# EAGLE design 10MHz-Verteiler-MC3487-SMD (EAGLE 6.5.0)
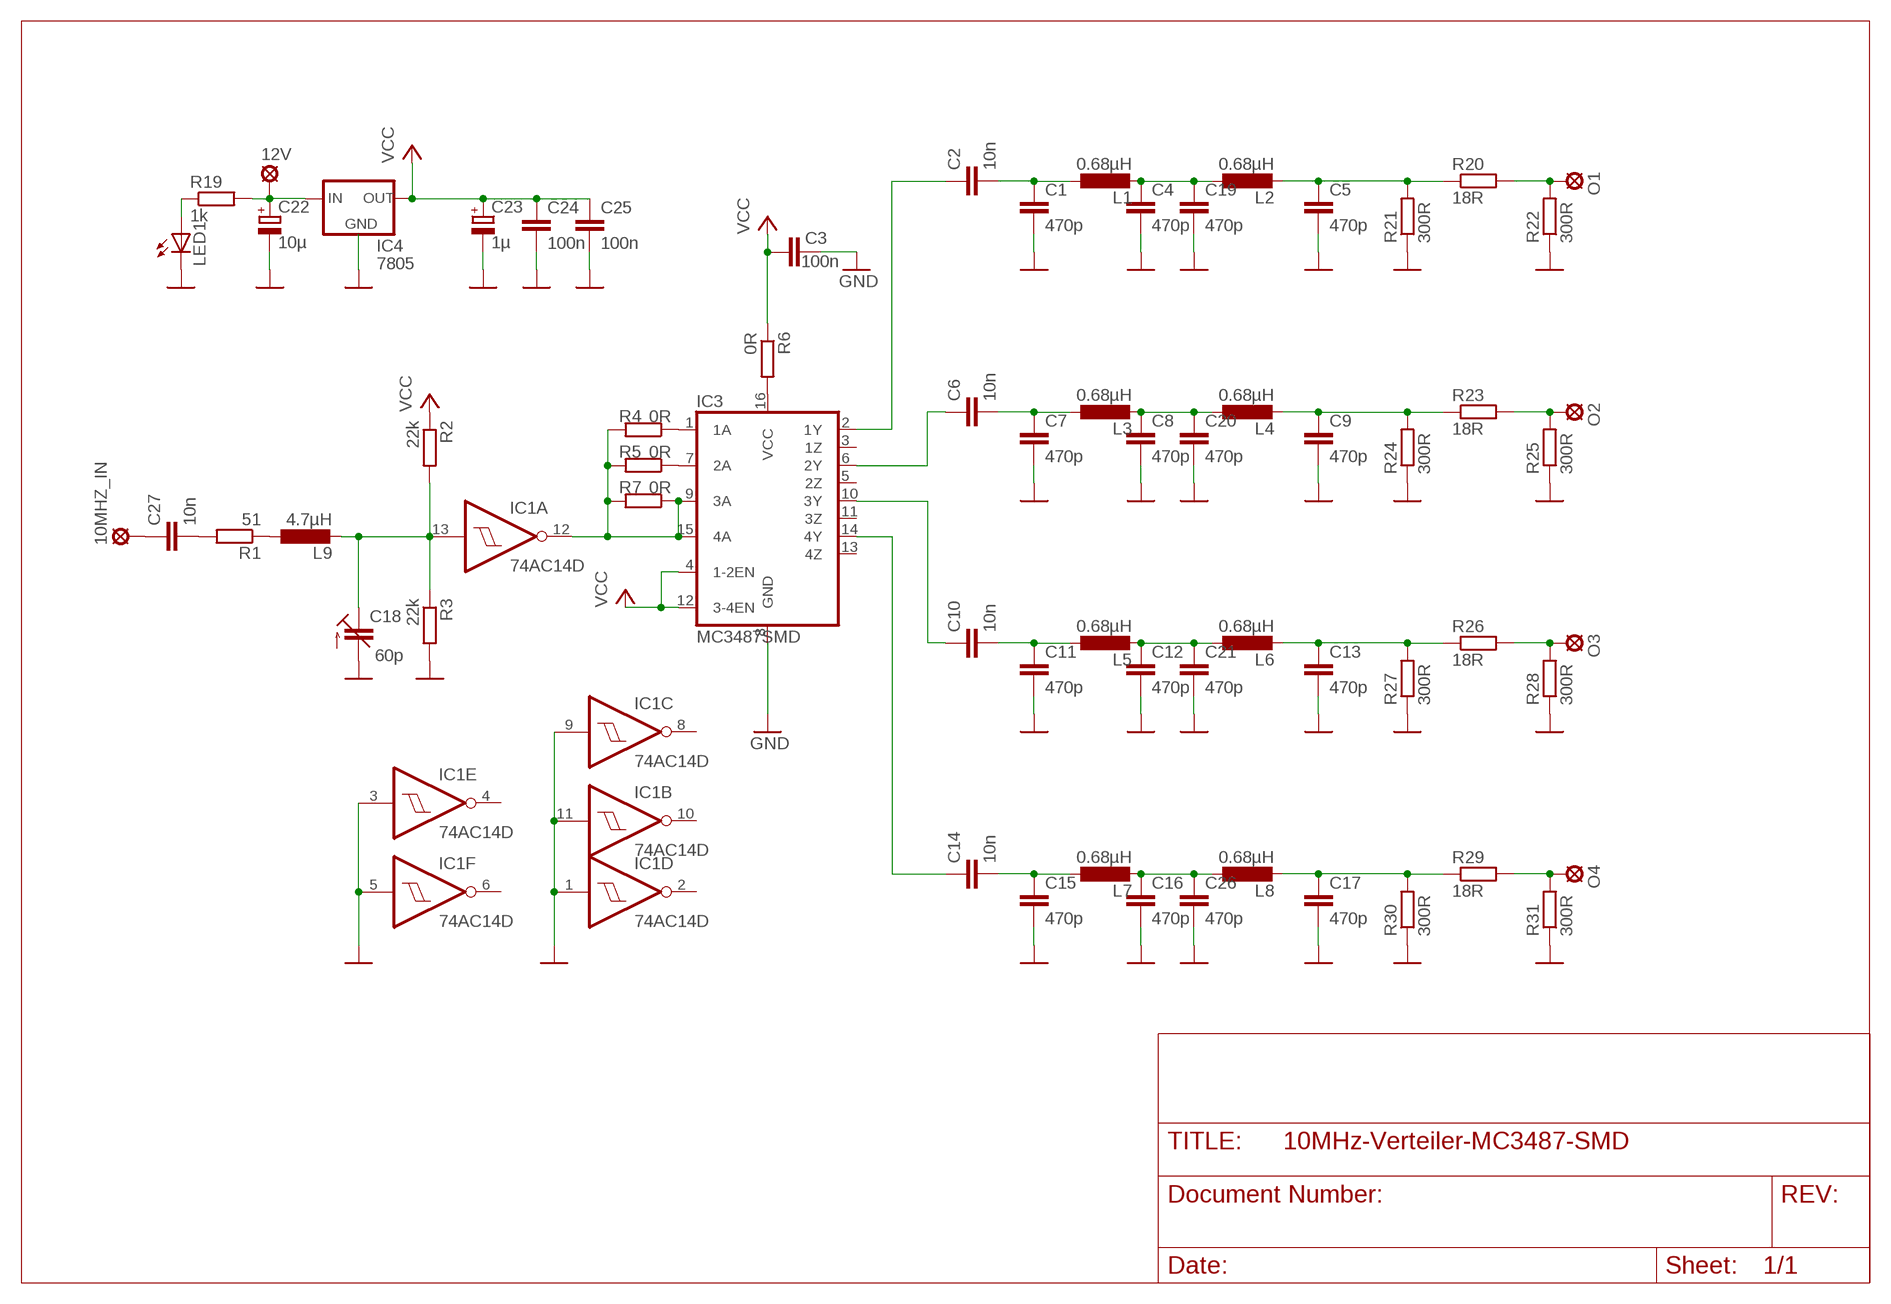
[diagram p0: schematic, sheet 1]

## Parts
10MHZ_IN  LSP10  [LSP10]
12V  LSP10  [LSP10]
C1  470p  C-EUC1206  [C1206]
C2  10n  C-EUC1206  [C1206]
C3  100n  C-EUC1206  [C1206]
C4  470p  C-EUC1206  [C1206]
C5  470p  C-EUC1206  [C1206]
C6  10n  C-EUC1206  [C1206]
C7  470p  C-EUC1206  [C1206]
C8  470p  C-EUC1206  [C1206]
C9  470p  C-EUC1206  [C1206]
C10  10n  C-EUC1206  [C1206]
C11  470p  C-EUC1206  [C1206]
C12  470p  C-EUC1206  [C1206]
C13  470p  C-EUC1206  [C1206]
C14  10n  C-EUC1206  [C1206]
C15  470p  C-EUC1206  [C1206]
C16  470p  C-EUC1206  [C1206]
C17  470p  C-EUC1206  [C1206]
C18  60p  C-TRIMM3018_12  [CTRIM3018_12]
C19  470p  C-EUC1206  [C1206]
C20  470p  C-EUC1206  [C1206]
C21  470p  C-EUC1206  [C1206]
C22  10µ  CPOL-EU153CLV-0405  [153CLV-0405]
C23  1µ  CPOL-EU153CLV-0405  [153CLV-0405]
C24  100n  C-EUC1206  [C1206]
C25  100n  C-EUC1206  [C1206]
C26  470p  C-EUC1206  [C1206]
C27  10n  C-EUC1206  [C1206]
IC1  74AC14D  [SO14]
IC3  MC3487SMD  [SO16]
IC4  7805  78XXS  [78XXS]
L1  0.68µH  L-EUL3230M  [L3230M]
L2  0.68µH  L-EUL3230M  [L3230M]
L3  0.68µH  L-EUL3230M  [L3230M]
L4  0.68µH  L-EUL3230M  [L3230M]
L5  0.68µH  L-EUL3230M  [L3230M]
L6  0.68µH  L-EUL3230M  [L3230M]
L7  0.68µH  L-EUL3230M  [L3230M]
L8  0.68µH  L-EUL3230M  [L3230M]
L9  4.7µH  L-EUL3230M  [L3230M]
LED1  LED5MM  [LED5MM]
O1  LSP10  [LSP10]
O2  LSP10  [LSP10]
O3  LSP10  [LSP10]
O4  LSP10  [LSP10]
R1  51  R-EU_R1206  [R1206]
R2  22k  R-EU_R1206  [R1206]
R3  22k  R-EU_R1206  [R1206]
R4  0R  R-EU_R1206  [R1206]
R5  0R  R-EU_R1206  [R1206]
R6  0R  R-EU_R1206  [R1206]
R7  0R  R-EU_R1206  [R1206]
R19  1k  R-EU_R1206  [R1206]
R20  18R  R-EU_R1206  [R1206]
R21  300R  R-EU_R1206  [R1206]
R22  300R  R-EU_R1206  [R1206]
R23  18R  R-EU_R1206  [R1206]
R24  300R  R-EU_R1206  [R1206]
R25  300R  R-EU_R1206  [R1206]
R26  18R  R-EU_R1206  [R1206]
R27  300R  R-EU_R1206  [R1206]
R28  300R  R-EU_R1206  [R1206]
R29  18R  R-EU_R1206  [R1206]
R30  300R  R-EU_R1206  [R1206]
R31  300R  R-EU_R1206  [R1206]

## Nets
GND: C1.2 C3.1 C4.2 C5.2 C7.2 C8.2 C9.2 C11.2 C12.2 C13.2 C15.2 C16.2 C17.2 C18.-(A) C19.2 C20.2 C21.2 C22.- C23.- C24.2 C25.2 C26.2 IC1.1(D:I) IC1.3(E:I) IC1.5(F:I) IC1.9(C:I) IC1.11(B:I) IC3.8(GND) IC4.GND LED1.K(C) R3.2 R21.1 R22.1 R24.1 R25.1 R27.1 R28.1 R30.1 R31.1 ; supply symbol labelled 
N$1: C14.1 IC3.14(4Y)
N$2: C1.1 C2.2 L1.1
N$3: C4.1 C19.1 L1.2 L2.1
N$4: IC1.12(A:O) IC3.9(3A) IC3.15(4A) R4.2 R5.2 R7.1 R7.2
N$5: C12.1 C21.1 L5.2 L6.1
N$6: C16.1 C26.1 L7.2 L8.1
N$7: C6.2 C7.1 L3.1
N$8: C8.1 C20.1 L3.2 L4.1
N$9: C9.1 L4.2 R23.1 R24.2
N$10: C5.1 L2.2 R20.1 R21.2
N$11: C2.1 IC3.2(1Y)
N$12: C10.2 C11.1 L5.1
N$13: 12V.MP C22.+ IC4.IN R19.2
N$14: C10.1 IC3.10(3Y)
N$15: C13.1 L6.2 R26.1 R27.2
N$16: C6.1 IC3.6(2Y)
N$17: C14.2 C15.1 L7.1
N$18: IC3.1(1A) R4.1
N$19: IC3.7(2A) R5.1
N$20: C17.1 L8.2 R29.1 R30.2
N$21: C27.2 R1.2
N$22: IC3.16(VCC) R6.2
N$23: 10MHZ_IN.MP C27.1
N$27: C18.+(E) IC1.13(A:I) L9.2 R2.2 R3.1
N$29: L9.1 R1.1
N$41: LED1.A R19.1
N$43: O1.MP R20.2 R22.2
N$44: O2.MP R23.2 R25.2
N$45: O3.MP R26.2 R28.2
N$47: O4.MP R29.2 R31.2
VCC: C3.2 C23.+ C24.1 C25.1 IC3.4(1-2EN) IC3.12(3-4EN) IC4.OUT R2.1 R6.1
Unconnected: IC1.2(D:O) IC1.4(E:O) IC1.6(F:O) IC1.8(C:O) IC1.10(B:O) IC3.3(1Z) IC3.5(2Z) IC3.11(3Z) IC3.13(4Z)

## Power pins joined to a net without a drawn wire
GND: IC1.7(P:GND)
VCC: IC1.14(P:VCC)

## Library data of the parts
10MHZ_IN 12V O1-O4 = solpad:LSP10: SOLDER PAD
C1-C17 C19-C21 C24-C27 = rcl:C-EU: CAPACITOR, European symbol
C18 = rcl:C-TRIMM: Trimm capacitor
C22 C23 = rcl:CPOL-EU: POLARIZED CAPACITOR, European symbol
IC1 = 74xx-eu:74*14: Hex schmitt trigger INVERTER
IC3 = dk3ha-2015-01:MC3487SMD
IC4 = v-reg:78XXS: VOLTAGE REGULATOR
L1-L9 = rcl:L-EU: INDUCTOR, European symbol
LED1 = led:LED: LED
R1-R7 R19-R31 = rcl:R-EU_: RESISTOR, European symbol

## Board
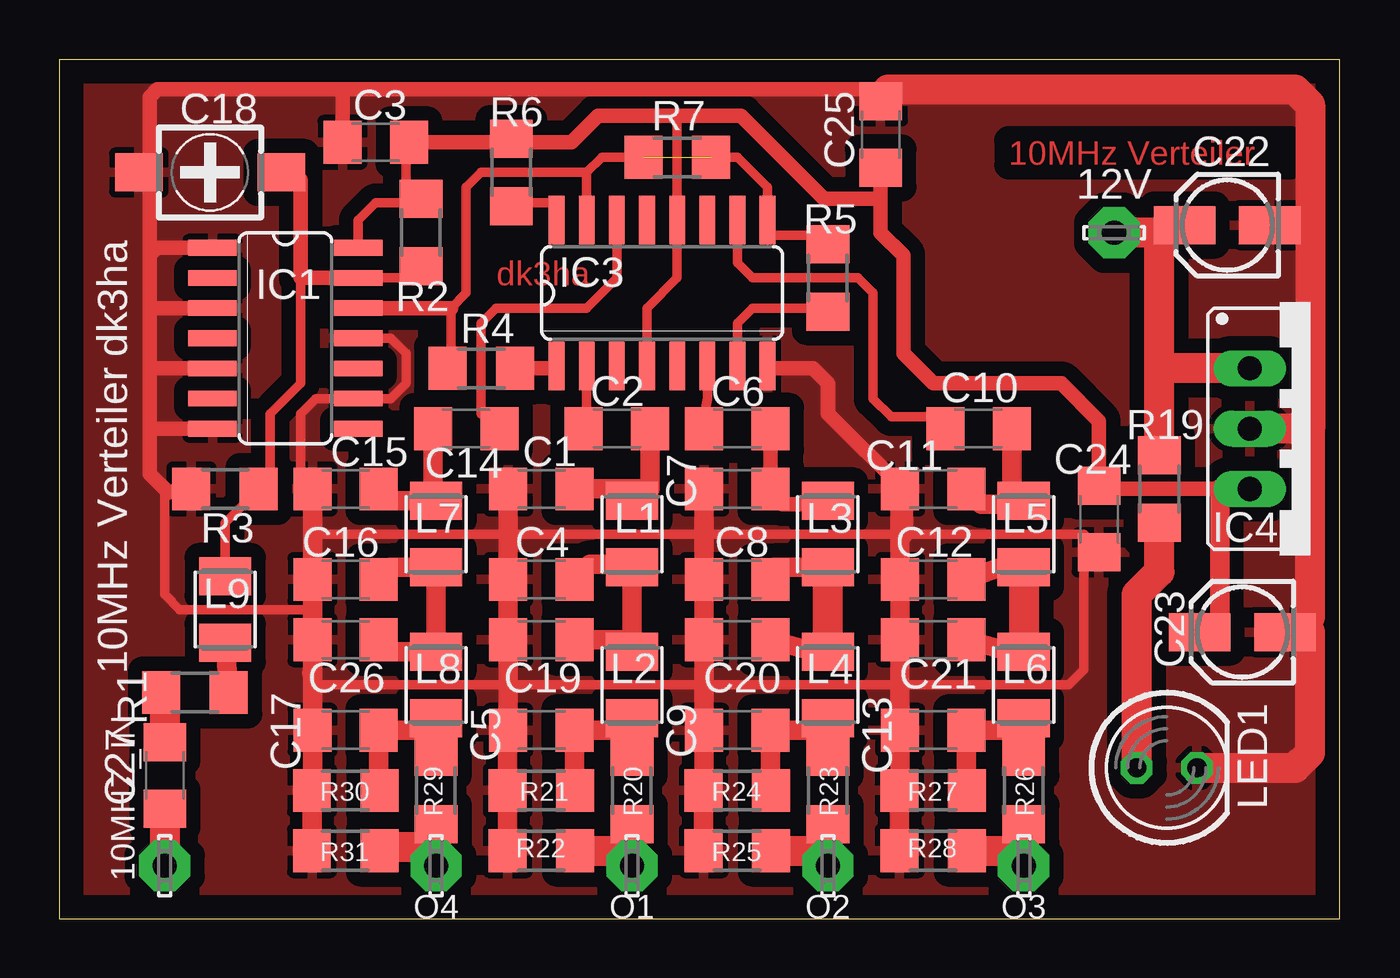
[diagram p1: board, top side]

Size 53.95 x 36.18 mm. Coordinates in mm from the lower left corner, seen from the top.
Outline: 0,0 53.95,0 53.95,36.18 0,36.18 0,0
Copper layers (1*16): Top 0.035mm / dielectric 1.5mm / Bottom 0.035mm
Design rules "default": minimum track width 10mil, minimum drill 24mil, track to track 8mil, track to pad 8mil, pad to pad 8mil, via to via 8mil, smd to smd 8mil, copper to edge 40mil, drill to drill 8mil, minimum pad ring 10mil, minimum via ring 8mil, stop-mask expansion 4mil, vias tented up to drill 0mil, thermal gap 10mil

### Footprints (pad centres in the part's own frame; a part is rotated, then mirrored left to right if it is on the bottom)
LSP10 = drill 1.016 pad 2.159 octagon: MP 0,0
C1206 = smd 1.6 x 1.8: 1 -1.4,0; 2 1.4,0
CTRIM3018_12 = smd 2 x 1.6: + -3,0; - 3,0
153CLV-0405 = smd 2.6 x 1.6: + 1.8,0; - -1.8,0
SO14 = smd 0.66 x 2.032: 1 -3.81,-3.073; 2 -2.54,-3.073; 3 -1.27,-3.073; 4 0,-3.073; 5 1.27,-3.073; 6 2.54,-3.073; 7 3.81,-3.073; 8 3.81,3.073; 9 2.54,3.073; 10 1.27,3.073; 11 0,3.073; 12 -1.27,3.073; 13 -2.54,3.073; 14 -3.81,3.073
SO16 = smd 0.66 x 2.032: 1 -3.175,-3.073; 2 -1.905,-3.073; 3 -0.635,-3.073; 4 0.635,-3.073; 5 1.905,-3.073; 6 3.175,-3.073; 7 4.445,-3.073; 8 5.715,-3.073; 9 5.715,3.073; 10 4.445,3.073; 11 3.175,3.073; 12 1.905,3.073; 13 0.635,3.073; 14 -0.635,3.073; 15 -1.905,3.073; 16 -3.175,3.073
78XXS = drill 1.016 long: GND 0,-2.54; IN -2.54,-2.54; OUT 2.54,-2.54
L3230M = smd 1.6 x 2.2: 1 -1.4,0; 2 1.4,0
LED5MM = drill 0.813 octagon: A -1.27,0; K 1.27,0
R1206 = smd 1.6 x 1.803: 1 -1.422,0; 2 1.422,0

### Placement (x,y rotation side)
10MHZ_IN  4.45,2.22 90 top
12V  44.45,28.89 0 top
C1  20.32,18.1 180 top
C2  23.5,20.64 0 top
C3  13.34,32.7 0 top
C4  20.32,14.29 180 top
C5  20.32,7.94 180 top
C6  28.57,20.64 0 top
C7  28.57,18.1 180 top
C8  28.57,14.29 180 top
C9  28.57,7.94 180 top
C10  38.73,20.64 0 top
C11  36.83,18.1 180 top
C12  36.83,14.29 180 top
C13  36.83,7.94 180 top
C14  17.14,20.64 180 top
C15  12.06,18.1 180 top
C16  12.06,14.29 180 top
C17  12.06,7.94 180 top
C18  6.35,31.43 180 top
C19  20.32,11.75 180 top
C20  28.57,11.75 180 top
C21  36.83,11.75 180 top
C22  49.21,29.21 180 top
C23  49.85,12.06 180 top
C24  43.81,16.83 270 top
C25  34.61,33.02 90 top
C26  12.06,11.75 180 top
C27  4.45,6.03 90 top
IC1  9.53,24.45 270 top
IC3  24.13,26.35 0 top
IC4  52.7,20.64 270 top
L1  24.13,16.19 270 top
L2  24.13,9.84 270 top
L3  32.38,16.19 270 top
L4  32.38,9.84 270 top
L5  40.64,16.19 270 top
L6  40.64,9.84 270 top
L7  15.88,16.19 270 top
L8  15.88,9.84 270 top
L9  6.99,13.02 90 top
LED1  46.67,6.35 0 top
O1  24.13,2.22 270 top
O2  32.38,2.22 270 top
O3  40.64,2.22 270 top
O4  15.88,2.22 270 top
R1  5.71,9.53 180 top
R2  15.24,28.89 270 top
R3  6.99,18.1 180 top
R4  17.78,23.18 180 top
R5  32.38,26.99 90 top
R6  19.05,31.43 270 top
R7  26.04,32.07 180 top
R19  46.35,18.1 90 top
R20  24.13,5.4 270 top
R21  20.32,5.4 0 top
R22  20.32,2.86 0 top
R23  32.38,5.4 270 top
R24  28.57,5.4 0 top
R25  28.57,2.86 0 top
R26  40.64,5.4 270 top
R27  36.83,5.4 0 top
R28  36.83,2.86 0 top
R29  15.88,5.4 270 top
R30  12.06,5.4 0 top
R31  12.06,2.86 0 top

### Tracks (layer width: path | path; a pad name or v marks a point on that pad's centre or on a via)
GND
  Top 0.406: 10.66,16.19 10.79,16.19 | 10.79,16.19 35.56,16.19 43.18,16.19 | 10.66,10.48 10.66,9.97 10.79,9.84 18.92,9.84 27.18,9.84 42.55,9.84 43.18,10.48 43.18,16.19 | 10.64,16.04 10.79,16.19 | R3.2 4.75,18.1 4.6,17.95 | 4.45,18.1 4.45,13.65 5.08,13.02 10.79,13.02 10.79,11.75 C26.2 | C24.2 43.18,16.19 | IC1.11 13.97,24.45 14.61,23.81 14.61,22.54 13.97,21.91 IC1.9 10.79,21.91 10.16,21.27 10.16,18.1 C15.2
  Top 0.61: 10.66,5.42 R30.1 | 10.79,2.71 R31.1 | 18.9,8.55 C5.2 | 27.18,5.42 R24.1 | 35.43,5.42 R27.1 | C11.2 35.56,17.59 35.56,18.1 32.38,21.27 32.38,22.54 31.75,23.18 29.95,23.18 IC3.8 | 3.81,25.72 3.81,23.18 | 3.81,23.18 3.81,20.64 | 3.81,20.64 IC1.7 | IC1.3 3.81,25.72 | IC1.5 3.81,23.18 | 10.54,10.35 10.66,10.48 | 4.6,17.95 4.45,18.1 3.81,18.73 3.81,20.64 | 3.81,25.72 3.81,27.94 | 3.81,27.94 3.81,30.97 3.74,31.04 | 3.74,31.04 C18.- | IC1.1 4.13,28.26 3.81,27.94 | 3.74,31.04 3.81,31.11 3.81,34.61 4.13,34.92 12.06,34.92 | 12.06,34.92 34.92,34.92 34.61,34.61 C25.2 | C3.1 11.94,34.8 12.06,34.92 | C22.- 52.7,29.21 | C23.- 52.07,12.06 52.39,11.75 | 52.39,11.75 52.7,12.06 52.7,12.7 52.39,11.75
  Top 0.813: C15.2 10.66,16.19 C16.2 C26.2 10.66,10.48 C17.2 10.66,5.42 | R30.1 R31.1 | R22.1 R21.1 18.9,8.55 | C5.2 18.92,9.84 C19.2 C4.2 C1.2 | C7.2 C8.2 C20.2 27.18,9.84 C9.2 27.18,5.42 | R24.1 R25.1 | C11.2 C12.2 C21.2 C13.2 35.43,5.42 | R27.1 R28.1 | 35.56,17.59 35.56,16.19
  Top 1.27: 34.92,34.92 52.07,34.92 52.7,34.29 52.7,29.21 52.7,20.64 | 52.7,20.64 IC4.GND | 52.7,12.7 52.7,20.64 | LED1.K 52.07,6.35 52.7,6.99 52.7,12.06
  pour Top (isolate 0.61): 0,36.04 54.13,36.04 53.98,0 -0.16,0
N$1
  Top 0.406: IC3.14 23.5,26.99 22.23,25.72 18.41,25.72 17.78,25.08 17.78,21.27 18.41,20.64 18.41,20.51 C14.1
N$2
  Top 0.61: 24.89,18.1 24.26,17.72
  Top 0.813: C2.2 24.89,18.1 C1.1 | 24.26,17.72 L1.1
N$3
  Top 0.61: 24,11.11 L2.1 | 24,14.92 L1.2
  Top 0.813: L1.2 L2.1 23.62,11.75 C19.1 | 24,14.92 22.36,14.92 C4.1
N$4  (1 unrouted)
  Top 0.406: 22.23,31.43 17.78,31.43 17.14,30.8 17.14,26.35 16.51,25.72 16.51,23.33 | 22.23,31.43 IC3.15 | R5.2 33.02,28.89 31.85,28.79 30.06,28.79 29.84,28.57 IC3.9 29.84,30.8 28.57,32.07 R7.1 | R7.2 22.86,32.07 22.23,31.43
  Top 0.61: 16.51,23.33 R4.2 | IC1.12 16.51,25.72
N$5
  Top 0.61: 40.51,11.11 L6.1 | 40.01,14.92 40.64,14.29
  Top 0.813: L5.2 40.64,14.29 | C21.1 40.51,11.11 | C12.1 40.01,14.92
  Top 1.27: 40.64,14.29 L6.1
N$6
  Top 0.813: C26.1 13.6,11.24 L8.1 L7.2 13.97,14.79 C16.1
N$7
  Top 0.61: L3.1 32.38,17.46 30.48,17.46 | C7.1 30.48,17.46 | C6.2 29.98,17.97 30.48,17.46
N$8
  Top 0.813: L3.2 30.11,14.79 C8.1 | C20.1 32.26,11.11 L4.1
  Top 1.27: L4.1 L3.2
N$9
  Top 0.61: 32.26,7.94 L4.2 | R24.2 29.98,5.4
  Top 0.813: R23.1 L4.2 | 32.26,7.94 C9.1 29.98,5.4
N$10
  Top 0.61: L2.2 24.13,7.94 | R21.2 21.72,5.4
  Top 0.813: R20.1 24.13,7.94 C5.1 21.72,5.4
N$11
  Top 0.406: IC3.2 22.23,21.27 21.59,20.64 21.59,20.13 C2.1
N$12
  Top 0.61: 40.51,17.46 L5.1 | 40.51,17.46 40.64,17.46 | 40.51,17.46 40.01,17.46 40.13,17.59
  Top 0.813: 40.01,17.46 38.87,17.46 C11.1 | C10.2 40.13,17.59
N$13
  Top 0.61: 46.35,28.89 46.35,29.21 C22.+ | 46.67,23.18 46.35,22.86
  Top 1.27: R19.2 46.35,22.86 46.35,28.89 12V.MP | IC4.IN 46.67,23.18
N$14
  Top 0.406: IC3.10 28.57,27.62 29.21,26.99 33.66,26.99 34.29,26.35 34.29,21.91 35.05,21.14 36.83,21.14 C10.1
N$15
  Top 0.61: L6.2 40.64,7.94 | R27.2 38.23,5.4
  Top 0.813: R26.1 40.64,7.94 C13.1 38.23,5.4
N$16
  Top 0.406: C6.1 27.18,21.14 27.3,21.91 IC3.6
N$17
  Top 0.61: L7.1 15.24,17.59 15.74,17.72
  Top 0.813: 15.24,17.59 13.97,17.59 C15.1 | C14.2 15.74,17.72
N$18
  Top 0.61: R4.1 20.85,23.18 IC3.1
N$19
  Top 0.406: IC3.7 28.57,25.08 29.21,25.72 32.87,25.72 R5.1
N$20
  Top 0.61: 15.88,7.94 L8.2 | R30.2 13.46,5.4
  Top 0.813: R29.1 15.88,7.94 C17.1 13.46,5.4
N$21
  Top 0.406: R1.2 4.45,9.53
  Top 1.27: 4.45,9.53 C27.2
N$22
  Top 0.406: R6.2 19.05,30.16 20.95,30.16 IC3.16
N$23
  Top 1.27: C27.1 10MHZ_IN.MP
N$27
  Top 0.406: R2.2 15.24,26.99 IC1.13 | 10.16,26.99 10.16,22.54 8.89,21.27 8.89,18.73 8.41,18.25 R3.1 6.99,16.68 L9.2
  Top 0.61: IC1.13 10.16,26.99 10.16,31.11 9.67,31.11 C18.+
N$29
  Top 0.813: L9.1 R1.1
N$41
  Top 1.27: LED1.A 45.4,13.65 46.35,14.61 R19.1
N$43
  Top 0.61: R20.2 O1.MP
  Top 1.27: R22.2 23.98,2.86 R20.2
N$44
  Top 0.61: 32.23,2.86 R23.2
  Top 1.27: O2.MP R23.2 | R25.2 32.23,2.86
N$45
  Top 0.61: 40.49,2.86 R26.2
  Top 1.27: R26.2 O3.MP | R28.2 40.49,2.86
N$47
  Top 0.61: 13.64,3.02 R31.2 | 15.88,3.02 O4.MP
  Top 1.27: R29.2 15.88,3.02 13.64,3.02
VCC
  Top 0.406: IC3.4 24.77,25.72 26.04,26.99 IC3.12 26.04,33.81 | 18.9,32.7 R6.1 | 15.24,32.7 14.61,33.34 14.61,32.07 | 14.61,32.07 14.61,30.16 | 14.61,30.16 15.09,30.16 R2.1 | C3.2 14.61,32.07 | IC1.14 12.6,29.43 13.34,30.16 14.61,30.16
  Top 0.61: 15.24,32.7 18.9,32.7 21.59,32.7 22.7,33.81 26.04,33.81 28.73,33.81 32.23,30.32 34.45,30.32 34.61,30.16 | IC4.OUT 48.9,18.1 43.95,18.1 C24.1 43.81,20.95 42.23,22.54 36.83,22.54 35.56,23.81 35.56,27.94 34.61,28.89 34.61,30.16 | 34.61,30.16 C25.1 | C23.+ 48.9,12.7
  Top 0.813: 48.9,12.7 48.9,18.1

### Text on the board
Top: 10MHz Verteiler | dk3ha
tPlace: dk3ha | 10MHz Verteiler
